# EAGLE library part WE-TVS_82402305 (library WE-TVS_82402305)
TVS Diode Array WE-TVS, Standard Series - Low capazity - No leakage current - Low clamping voltage - high ESD voltage protection - Uni- and bidirectional protection -- DC Distribution -- Headsets and Accessoires -- PDAs -- Digital Cameras -- MP3-Players -- Touch Panels
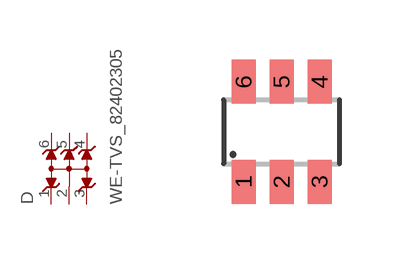
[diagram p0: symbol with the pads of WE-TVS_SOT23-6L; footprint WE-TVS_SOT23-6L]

Designator prefix D

## WE-TVS_82402305 (MPN: 82402305; OC_FARNELL: 1825866; OC_NEWARK: 79R6955; PACKAGE: SOT23-6L; SUPPLIER: Wuerth Elektronik)  [WE-TVS_SOT23-6L]
1  1  pas
2  GND  pwr
3  2  pas
4  3  pas
5  4  pas
6  5  pas

## Footprint WE-TVS_SOT23-6L (pad centres in mm)
TVS Diode Array WE-TVS
smd 0.6 x 1.1: 1 -0.95,-1.25; 2 0,-1.25; 3 0.95,-1.25; 4 0.95,1.25; 5 0,1.25; 6 -0.95,1.25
